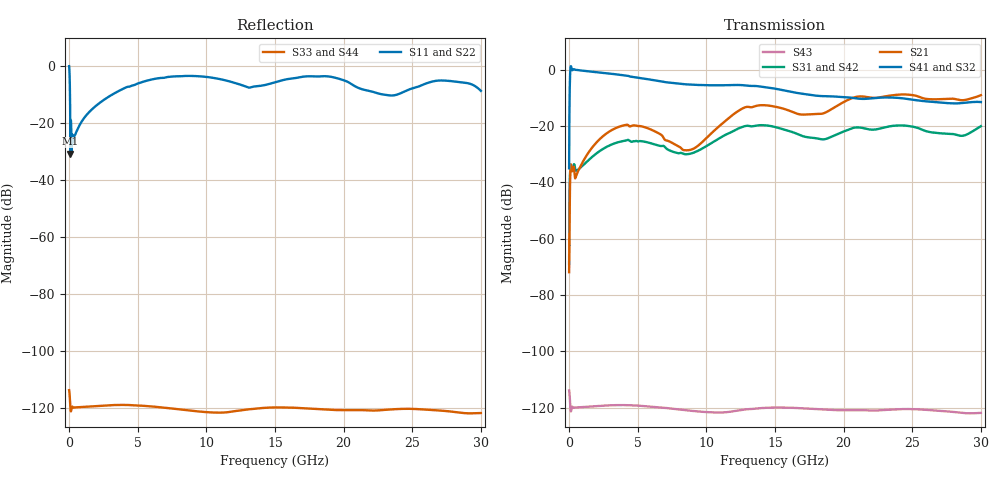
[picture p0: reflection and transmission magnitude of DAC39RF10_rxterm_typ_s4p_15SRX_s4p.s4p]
! Touchstone generated by fitter/viewer
# HZ S  RI R 5.000000e+01
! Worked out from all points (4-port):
!   3299 points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, 9.094 MHz to 30 GHz, reference 50 ohm
!   strongest paths, dB at 9.094 MHz, 7.502 GHz, 15 GHz, 22.51 GHz, 30 GHz:
!     S41: -35.0, -4.7, -6.7, -10.0, -11.5
!     S32: -35.0, -4.7, -6.7, -9.9, -11.5
!     S21: -71.9, -25.9, -13.1, -9.9, -9.0
!     S31: -69.0, -29.0, -20.3, -21.0, -20.0
!     S42: -69.1, -28.9, -20.4, -20.9, -20.0
!     S43: -113.8, -120.3, -119.9, -120.9, -121.8
!   lowest |S11| = -30.8 dB at 100 MHz (marker M1), VSWR 1.06, Z = 52.5 - j1.51 ohm
!   |S11| at or under -10 dB: 72.33 MHz to 3.188 GHz (3.116 GHz wide, 191 % of centre); 22.76 GHz to 23.98 GHz (1.212 GHz wide, 5.19 % of centre)
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9093665  0.9828 0.000166  5.51e-06 0.000252  1.77e-08 -1.23e-09  1.77e-08 -1.23e-09
         5.57e-06 0.000255  0.9828 0.000148  1.77e-08 -1.22e-09  1.77e-08 -1.22e-09
         0.00032 -0.000154  0.0178 -0.000886  2.04e-06 -8.69e-09  2.04e-06 -8.69e-09
         0.0178 -0.00102  0.000321 -0.000146  2.04e-06 -8.69e-09  2.04e-06 -8.69e-09
1.000303e8  0.0249 -0.0143  0.0161 0.00279  9.95e-07 -4e-08  9.95e-07 -4e-08
            0.0161 0.00284  0.0251 -0.0146  9.95e-07 -3.96e-08  9.95e-07 -3.96e-08
            0.0159 -0.000107  1.019 -0.0529  1e-06 5.23e-09  1e-06 5.23e-09
            1.019 -0.0537  0.016 -8.94e-05  1e-06 4.91e-09  1e-06 4.91e-09
3.937557e9  0.1232 0.3744  0.1017 -0.00331  1.21e-07 -9.06e-07  1.21e-07 -9.06e-07
            0.1021 -0.00323  0.1235 0.3744  1.23e-07 -9.04e-07  1.23e-07 -9.04e-07
            -0.0528 0.012  -0.1385 -0.783  1.12e-06 -6.95e-08  1.12e-06 -6.95e-08
            -0.1382 -0.7859  -0.053 0.0119  1.12e-06 -6.99e-08  1.12e-06 -6.99e-08
8.611701e9  0.0256 -0.6632  -0.0349 -0.0116  -7.55e-07 -2.36e-07  -7.55e-07 -2.36e-07
            -0.0349 -0.0127  0.038 -0.6736  -7.52e-07 -2.43e-07  -7.52e-07 -2.43e-07
            0.0119 0.0293  -0.5269 0.1335  8.89e-07 -1.6e-07  8.89e-07 -1.6e-07
            -0.5306 0.1368  0.0121 0.0296  8.88e-07 -1.57e-07  8.88e-07 -1.57e-07
1.203092e10  -0.4393 0.2451  0.1222 0.111  -6.29e-07 7.17e-07  -6.29e-07 7.17e-07
             0.1214 0.1119  -0.4523 0.2229  -6.47e-07 7.02e-07  -6.47e-07 7.02e-07
             0.077 0.031  -0.0959 0.5225  8.67e-07 4.58e-08  8.67e-07 4.58e-08
             -0.0872 0.5286  0.0759 0.0316  8.74e-07 4.75e-08  8.74e-07 4.75e-08
1.508639e10  0.5111 -0.0963  -0.0137 -0.2197  4.12e-07 7.45e-07  4.12e-07 7.45e-07
             -0.0138 -0.2181  0.5048 -0.0993  4.08e-07 7.57e-07  4.08e-07 7.57e-07
             0.0226 -0.0924  0.3956 0.2282  1.01e-06 -1.35e-08  1.01e-06 -1.35e-08
             0.3974 0.226  0.0248 -0.0912  1.01e-06 -1.87e-08  1.01e-06 -1.87e-08
3e10  -0.347 -0.1055  0.1134 0.3348  -6e-07 5.02e-07  -6e-07 5.02e-07
      0.1126 0.3349  -0.3551 -0.1316  -6.3e-07 4.75e-07  -6.3e-07 4.75e-07
      0.0961 0.026  -0.1111 0.2433  8.08e-07 1.05e-08  8.08e-07 1.05e-08
      -0.1018 0.2461  0.0946 0.0312  8.14e-07 1.37e-08  8.14e-07 1.37e-08
